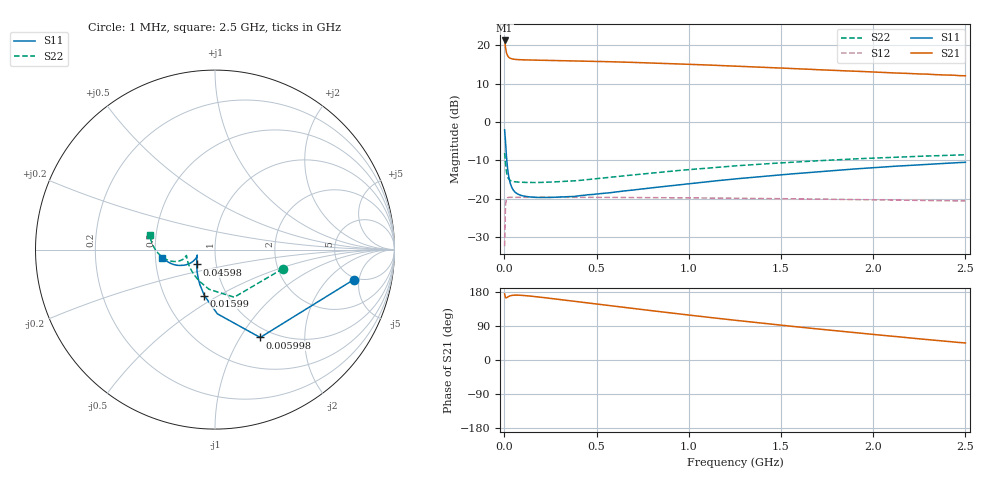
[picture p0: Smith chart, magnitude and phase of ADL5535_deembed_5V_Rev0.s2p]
!Agilent Technologies,N5230A,MY45000942,A.07.12.01
!Agilent N5230A: A.07.12.01
!Date: Thursday, January 07, 2010 10:57:54
!Correction: S11(Full 2 Port(1,2))
!S21(Full 2 Port(1,2))
!S12(Full 2 Port(1,2))
!S22(Full 2 Port(1,2))
!S2P File: Measurements: S11, S21, S12, S22:
# Hz S  dB  R 50
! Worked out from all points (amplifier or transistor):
!   501 points, 1 MHz to 2.5 GHz, reference 50 ohm
!   highest |S21| = 21.3 dB at 1 MHz (marker M1)
!   |S21| within 3 dB of that: start of sweep to 10.22 MHz
!   unconditionally stable (mu >= 1): 25.31 MHz to end of sweep
!   at 415.8 MHz: K = 1.07, MAG = 16.2 dB, |S12| = -19.7 dB
!   at 1.25 GHz: K = 1.06, MAG = 15.8 dB, |S12| = -19.9 dB
!   at 2.5 GHz: K = 1.15, MAG = 14.0 dB, |S12| = -20.6 dB
!   S11 on the Smith chart (normalised r, x): 1 MHz: 4.70, -4.20; 5.998 MHz: 0.87, -1.22; 15.99 MHz: 0.78, -0.43; 45.98 MHz: 0.80, -0.14; 2.5 GHz: 0.54, -0.05
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1000000  -2.04 -12.2  21.29 174.4  -32.45 45.9  -8.12 -15.7
5998000  -5.18 -62.8  19.41 164.3  -21.60 34.5  -10.87 -68.0
1.5994e7  -11.61 -103.1  17.41 165.8  -19.82 13.6  -14.14 -116.6
2.0992e7  -13.52 -113.8  17.03 167.3  -19.72 9.9  -14.73 -128.4
2.599e7  -14.88 -121.8  16.81 168.5  -19.69 7.5  -15.06 -136.6
3.5986e7  -16.63 -133.2  16.56 170.0  -19.68 4.7  -15.38 -147.1
4.5982e7  -17.63 -140.9  16.43 170.8  -19.68 3.1  -15.53 -153.4
7.597e7  -18.92 -153.4  16.28 171.1  -19.69 0.3  -15.72 -162.5
1.20952e8  -19.49 -160.3  16.20 169.6  -19.68 -2.2  -15.80 -167.2
2.85886e8  -19.65 -161.9  16.06 160.5  -19.67 -8.6  -15.64 -167.4
4.20832e8  -19.21 -158.1  15.90 152.5  -19.68 -13.3  -15.21 -164.8
6.45742e8  -18.05 -153.7  15.64 139.1  -19.73 -20.9  -14.09 -162.5
8.35666e8  -17.02 -151.8  15.34 128.0  -19.78 -27.2  -13.18 -162.6
1.015594e9  -16.04 -151.2  15.04 117.7  -19.84 -33.2  -12.37 -164.0
1.130548e9  -15.47 -151.6  14.83 111.4  -19.89 -37.0  -11.91 -165.5
1.2505e9  -14.89 -152.1  14.59 104.9  -19.93 -40.9  -11.48 -167.1
1.5004e9  -13.81 -154.3  14.09 92.0  -20.05 -49.0  -10.69 -171.3
1.670332e9  -13.13 -156.4  13.72 83.3  -20.13 -54.6  -10.22 -174.3
1.930228e9  -12.17 -160.4  13.20 70.7  -20.27 -63.1  -9.59 -179.7
2.085166e9  -11.67 -163.2  12.87 63.4  -20.37 -68.0  -9.27 176.9
2.305078e9  -11.04 -167.4  12.46 53.4  -20.52 -75.2  -8.88 171.9
2.5e9  -10.54 -171.4  12.06 45.0  -20.64 -81.5  -8.57 167.4
